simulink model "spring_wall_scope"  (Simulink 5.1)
settings: Solver=ode5  StartTime=0.0  StopTime=tfinal  FixedStep=Deltat  RelTol=1e-3
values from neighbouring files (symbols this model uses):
  B = 2*sqrt(20)    [prob1_PS5.m]
  K = 10    [prob1_PS5.m]
  M = 2    [prob1_PS5.m]
  z0 = 2    [prob1_PS5.m]
  z_w = 1    [prob1_PS5.m]

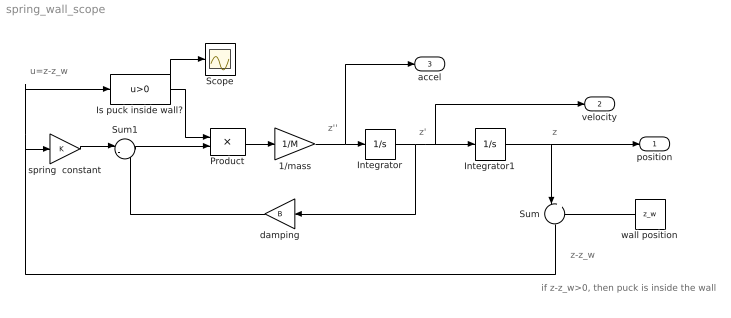
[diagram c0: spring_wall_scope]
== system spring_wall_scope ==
  note: z
  note: z'
  note: z''
  note: z-z_w
  note: if z-z_w>0, then puck is inside the wall
  note: u=z-z_w
  1/mass : Gain  Gain=1/M
  Integrator : Integrator
  Integrator1 : Integrator  InitialCondition=z0
  Is puck inside wall? : Fcn  Expr=u>0
  Product : Product
  Scope : Scope
  Sum : Sum  Orientation=down  Inputs=|+-
  Sum1 : Sum  Inputs=|--
  damping : Gain  Orientation=left  Gain=B
  spring  constant : Gain  Gain=K
  wall position : Constant  Orientation=left  Value=z_w
  position : Outport
  velocity : Outport  Port=2
  accel : Outport  Port=3
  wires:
  Integrator/1 -> damping/1, Integrator1/1, velocity/1
  Integrator1/1 -> position/1, Sum/1
  wall position/1 -> Sum/2
  Sum/1 -> spring  constant/1, Is puck inside wall?/1
  spring  constant/1 -> Sum1/1
  damping/1 -> Sum1/2
  Sum1/1 -> Product/2
  Is puck inside wall?/1 -> Product/1, Scope/1
  Product/1 -> 1/mass/1
  1/mass/1 -> Integrator/1, accel/1
